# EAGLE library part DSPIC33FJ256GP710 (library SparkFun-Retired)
Microchip 16-bit DSP SparkFun Products None Not tested
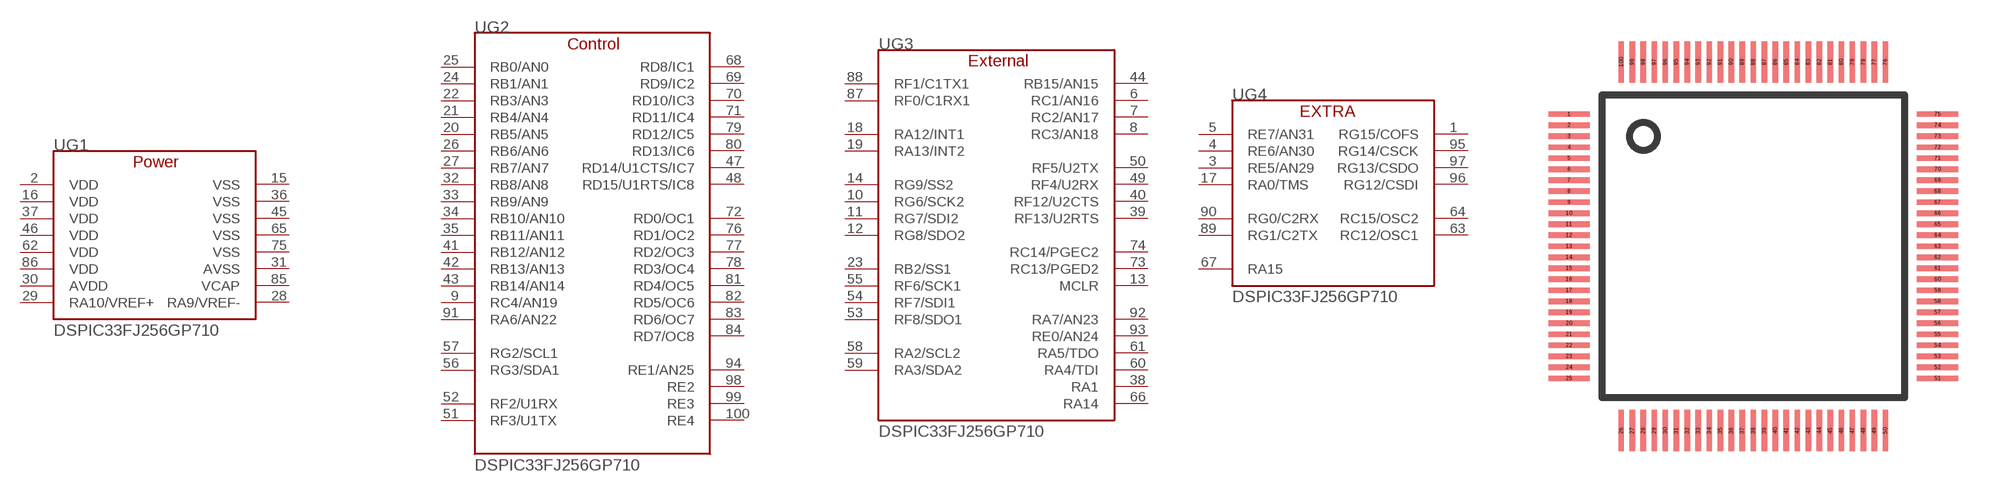
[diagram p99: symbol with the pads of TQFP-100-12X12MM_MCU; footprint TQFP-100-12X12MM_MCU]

Designator prefix U; gates G1=DSPIC33FJ256GP710_POWER G2=DSPIC33FJ256GP710_CONTROL G3=DSPIC33FJ256GP710_EXTERNAL G4=DSPIC33FJ256GP710_EXTRA

## DSPIC33FJ256GP710_  [TQFP-100-12X12MM_MCU]
1  G4:RG15/COFS
2  G1:VDD
3  G4:RE5/AN29
4  G4:RE6/AN30
5  G4:RE7/AN31
6  G3:RC1/AN16
7  G3:RC2/AN17
8  G3:RC3/AN18
9  G2:RC4/AN19
10  G3:RG6/SCK2
11  G3:RG7/SDI2
12  G3:RG8/SDO2
13  G3:MCLR
14  G3:RG9/SS2
15  G1:VSS
16  G1:VDD
17  G4:RA0/TMS
18  G3:RA12/INT1
19  G3:RA13/INT2
20  G2:RB5/AN5
21  G2:RB4/AN4
22  G2:RB3/AN3
23  G3:RB2/SS1
24  G2:RB1/AN1
25  G2:RB0/AN0
26  G2:RB6/AN6
27  G2:RB7/AN7
28  G1:RA9/VREF-
29  G1:RA10/VREF+
30  G1:AVDD
31  G1:AVSS
32  G2:RB8/AN8
33  G2:RB9/AN9
34  G2:RB10/AN10
35  G2:RB11/AN11
36  G1:VSS
37  G1:VDD
38  G3:RA1
39  G3:RF13/U2RTS
40  G3:RF12/U2CTS
41  G2:RB12/AN12
42  G2:RB13/AN13
43  G2:RB14/AN14
44  G3:RB15/AN15
45  G1:VSS
46  G1:VDD
47  G2:RD14/U1CTS/IC7
48  G2:RD15/U1RTS/IC8
49  G3:RF4/U2RX
50  G3:RF5/U2TX
51  G2:RF3/U1TX
52  G2:RF2/U1RX
53  G3:RF8/SDO1
54  G3:RF7/SDI1
55  G3:RF6/SCK1
56  G2:RG3/SDA1
57  G2:RG2/SCL1
58  G3:RA2/SCL2
59  G3:RA3/SDA2
60  G3:RA4/TDI
61  G3:RA5/TDO
62  G1:VDD
63  G4:RC12/OSC1
64  G4:RC15/OSC2
65  G1:VSS
66  G3:RA14
67  G4:RA15
68  G2:RD8/IC1
69  G2:RD9/IC2
70  G2:RD10/IC3
71  G2:RD11/IC4
72  G2:RD0/OC1
73  G3:RC13/PGED2
74  G3:RC14/PGEC2
75  G1:VSS
76  G2:RD1/OC2
77  G2:RD2/OC3
78  G2:RD3/OC4
79  G2:RD12/IC5
80  G2:RD13/IC6
81  G2:RD4/OC5
82  G2:RD5/OC6
83  G2:RD6/OC7
84  G2:RD7/OC8
85  G1:VCAP
86  G1:VDD
87  G3:RF0/C1RX1
88  G3:RF1/C1TX1
89  G4:RG1/C2TX
90  G4:RG0/C2RX
91  G2:RA6/AN22
92  G3:RA7/AN23
93  G3:RE0/AN24
94  G2:RE1/AN25
95  G4:RG14/CSCK
96  G4:RG12/CSDI
97  G4:RG13/CSDO
98  G2:RE2
99  G2:RE3
100  G2:RE4

## Footprint TQFP-100-12X12MM_MCU (pad centres in mm)
smd 1.5 x 0.2: 1 -6.7,4.8; 2 -6.7,4.4; 3 -6.7,4; 4 -6.7,3.6; 5 -6.7,3.2; 6 -6.7,2.8; 7 -6.7,2.4; 8 -6.7,2; 9 -6.7,1.6; 10 -6.7,1.2; 11 -6.7,0.8; 12 -6.7,0.4; 13 -6.7,0; 14 -6.7,-0.4; 15 -6.7,-0.8; 16 -6.7,-1.2; 17 -6.7,-1.6; 18 -6.7,-2; 19 -6.7,-2.4; 20 -6.7,-2.8; 21 -6.7,-3.2; 22 -6.7,-3.6; 23 -6.7,-4; 24 -6.7,-4.4; 25 -6.7,-4.8; 51 6.7,-4.8; 52 6.7,-4.4; 53 6.7,-4; 54 6.7,-3.6; 55 6.7,-3.2; 56 6.7,-2.8; 57 6.7,-2.4; 58 6.7,-2; 59 6.7,-1.6; 60 6.7,-1.2; 61 6.7,-0.8; 62 6.7,-0.4; 63 6.7,0; 64 6.7,0.4; 65 6.7,0.8; 66 6.7,1.2; 67 6.7,1.6; 68 6.7,2; 69 6.7,2.4; 70 6.7,2.8; 71 6.7,3.2; 72 6.7,3.6; 73 6.7,4; 74 6.7,4.4; 75 6.7,4.8
smd 0.2 x 1.5: 26 -4.8,-6.7; 27 -4.4,-6.7; 28 -4,-6.7; 29 -3.6,-6.7; 30 -3.2,-6.7; 31 -2.8,-6.7; 32 -2.4,-6.7; 33 -2,-6.7; 34 -1.6,-6.7; 35 -1.2,-6.7; 36 -0.8,-6.7; 37 -0.4,-6.7; 38 0,-6.7; 39 0.4,-6.7; 40 0.8,-6.7; 41 1.2,-6.7; 42 1.6,-6.7; 43 2,-6.7; 44 2.4,-6.7; 45 2.8,-6.7; 46 3.2,-6.7; 47 3.6,-6.7; 48 4,-6.7; 49 4.4,-6.7; 50 4.8,-6.7; 76 4.8,6.7; 77 4.4,6.7; 78 4,6.7; 79 3.6,6.7; 80 3.2,6.7; 81 2.8,6.7; 82 2.4,6.7; 83 2,6.7; 84 1.6,6.7; 85 1.2,6.7; 86 0.8,6.7; 87 0.4,6.7; 88 0,6.7; 89 -0.4,6.7; 90 -0.8,6.7; 91 -1.2,6.7; 92 -1.6,6.7; 93 -2,6.7; 94 -2.4,6.7; 95 -2.8,6.7; 96 -3.2,6.7; 97 -3.6,6.7; 98 -4,6.7; 99 -4.4,6.7; 100 -4.8,6.7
